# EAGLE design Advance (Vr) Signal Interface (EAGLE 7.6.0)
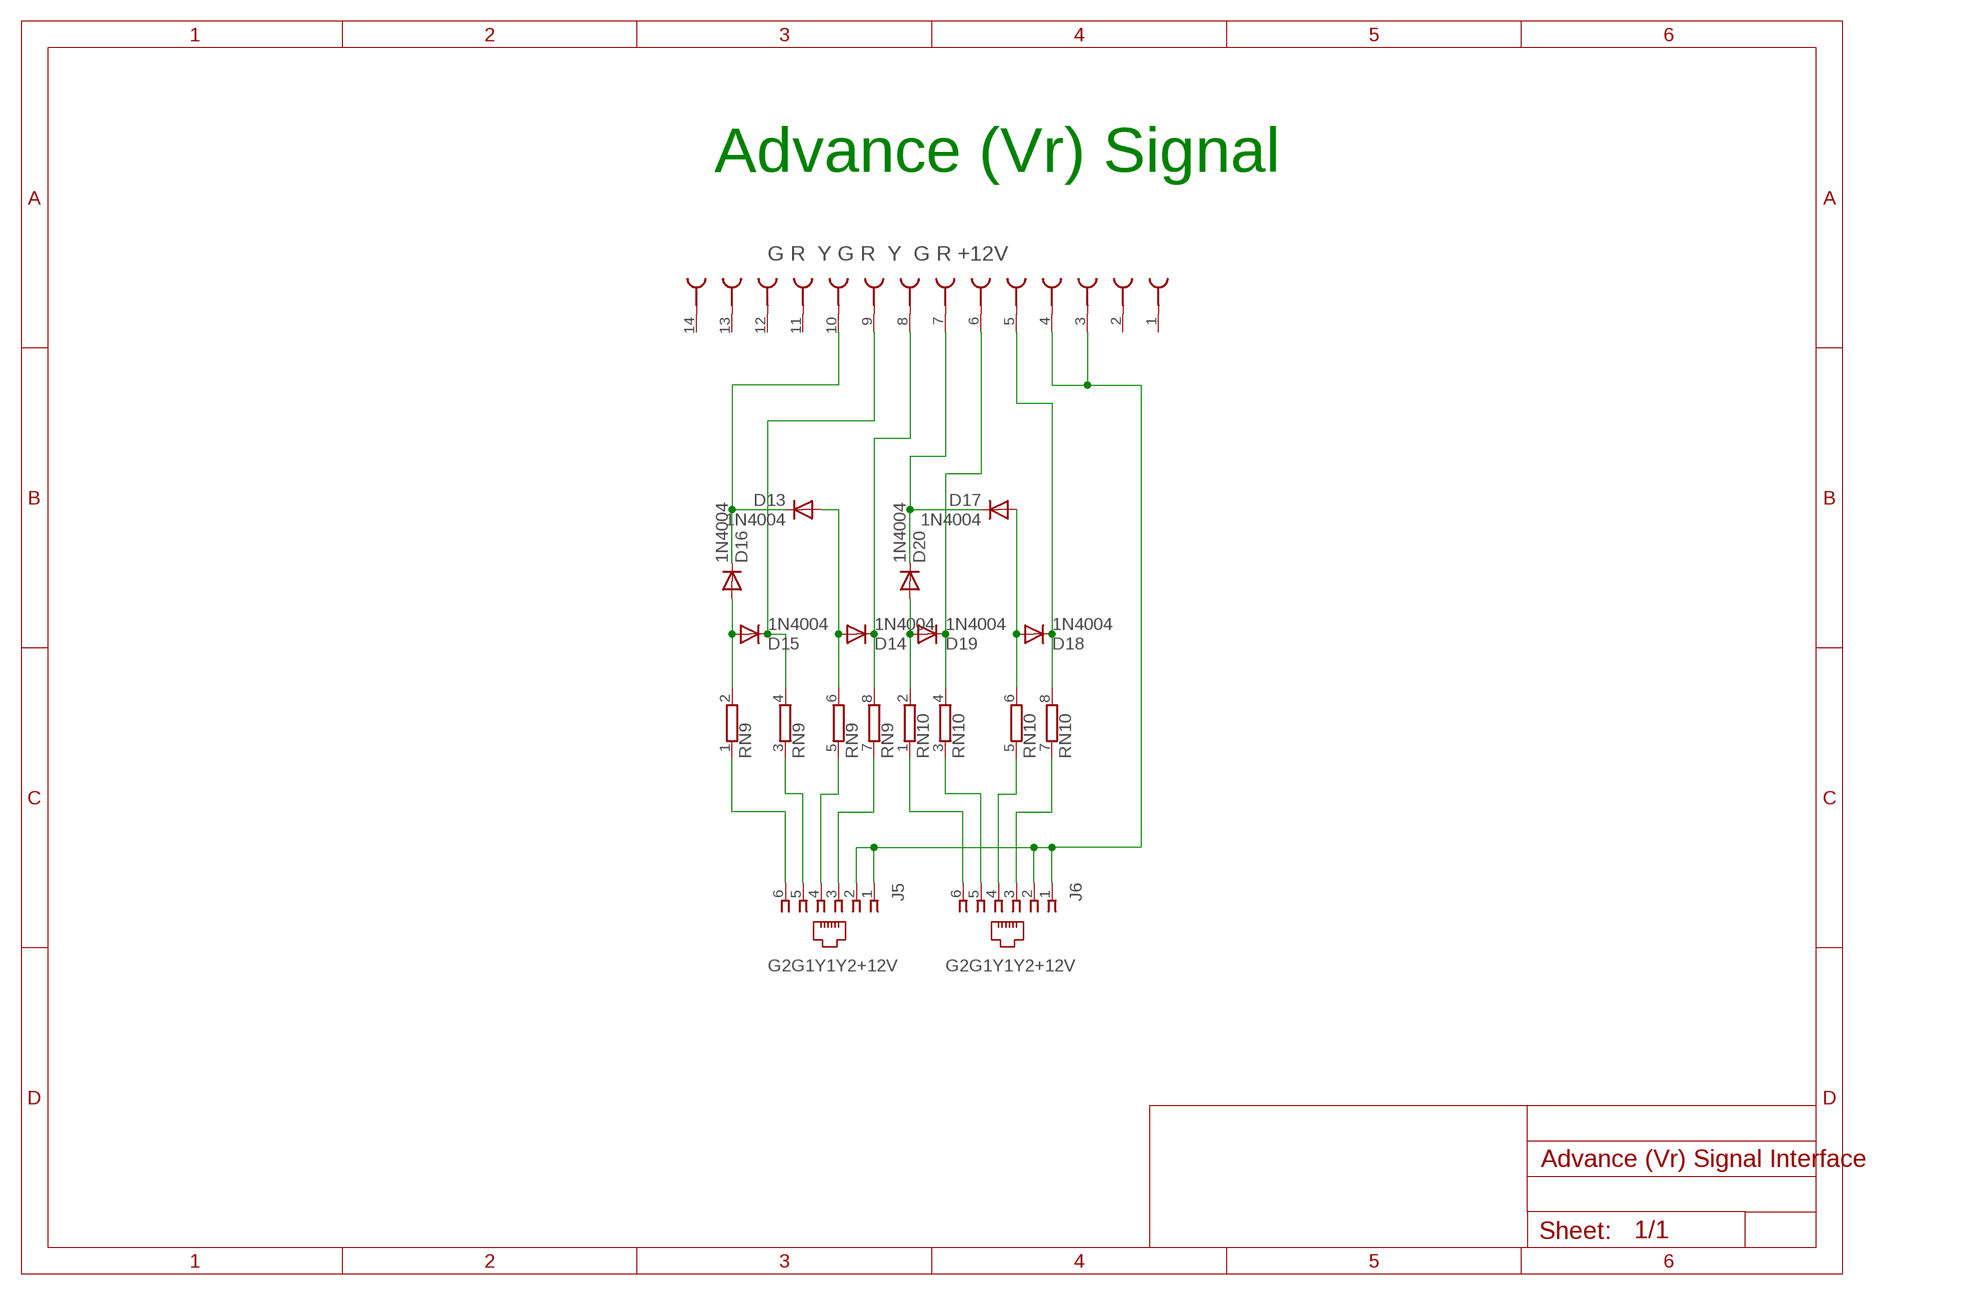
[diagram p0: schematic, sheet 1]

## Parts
D13  1N4004  [DO41-10]
D14  1N4004  [DO41-10]
D15  1N4004  [DO41-10]
D16  1N4004  [DO41-10]
D17  1N4004  [DO41-10]
D18  1N4004  [DO41-10]
D19  1N4004  [DO41-10]
D20  1N4004  [DO41-10]
J5  520250-3  [520250-3]
J6  520250-3  [520250-3]
RN9  E4RP  [SIL8]
RN10  E4RP  [SIL8]
U$11  AMP_FEMALE_PLUG  [AMP_FEMALE_PLUG]

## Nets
N$47: J5.3 RN9.7
N$48: D13.C D16.C U$11.10(SK9)
N$49: D13.A D14.A RN9.6
N$50: D15.A D16.A RN9.2
N$51: D14.C RN9.8 U$11.8(SK7)
N$52: D15.C RN9.4 U$11.9(SK8)
N$53: J5.4 RN9.5
N$54: J5.5 RN9.3
N$55: J5.6 RN9.1
N$56: J5.1 J5.2 J6.1 J6.2 U$11.3(SK2) U$11.4(SK3)
N$57: D18.C RN10.8 U$11.5(SK4)
N$58: J6.4 RN10.5
N$59: J6.5 RN10.3
N$60: J6.6 RN10.1
N$61: J6.3 RN10.7
N$62: D19.A D20.A RN10.2
N$63: D19.C RN10.4 U$11.6(SK5)
N$64: D17.C D20.C U$11.7(SK6)
N$84: D17.A D18.A RN10.6
Unconnected: U$11.1(SK) U$11.2(SK1) U$11.11(SK10) U$11.12(SK11) U$11.13(SK12) U$11.14(SK13)

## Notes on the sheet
- Advance (Vr) Signal
- G R  Y G R  Y  G R +12V
- G2G1Y1Y2+12V | G2G1Y1Y2+12V

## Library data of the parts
D13-D20 = diode:1N4004: DIODE
J5 J6 = con-amp:520250-3: AMP connector; MF: TYCO ELECTRONICS; MPN: 5520250-3; OC_FARNELL: unknown; OC_NEWARK: 42K8724
RN9 RN10 = resistor-sil:E4RP: SIL RESISTOR; OC_FARNELL: unknown; OC_NEWARK: unknown
U$11 = con-3m:AMP_FEMALE_PLUG

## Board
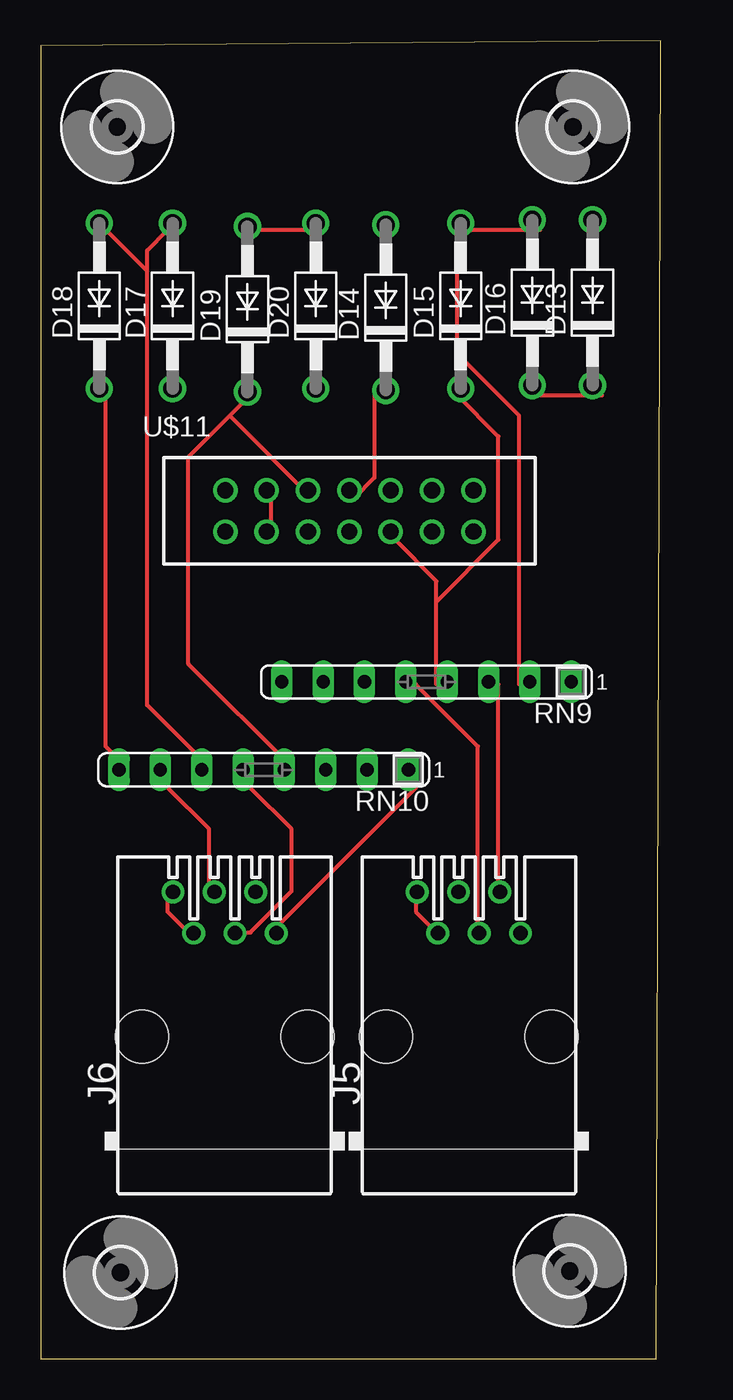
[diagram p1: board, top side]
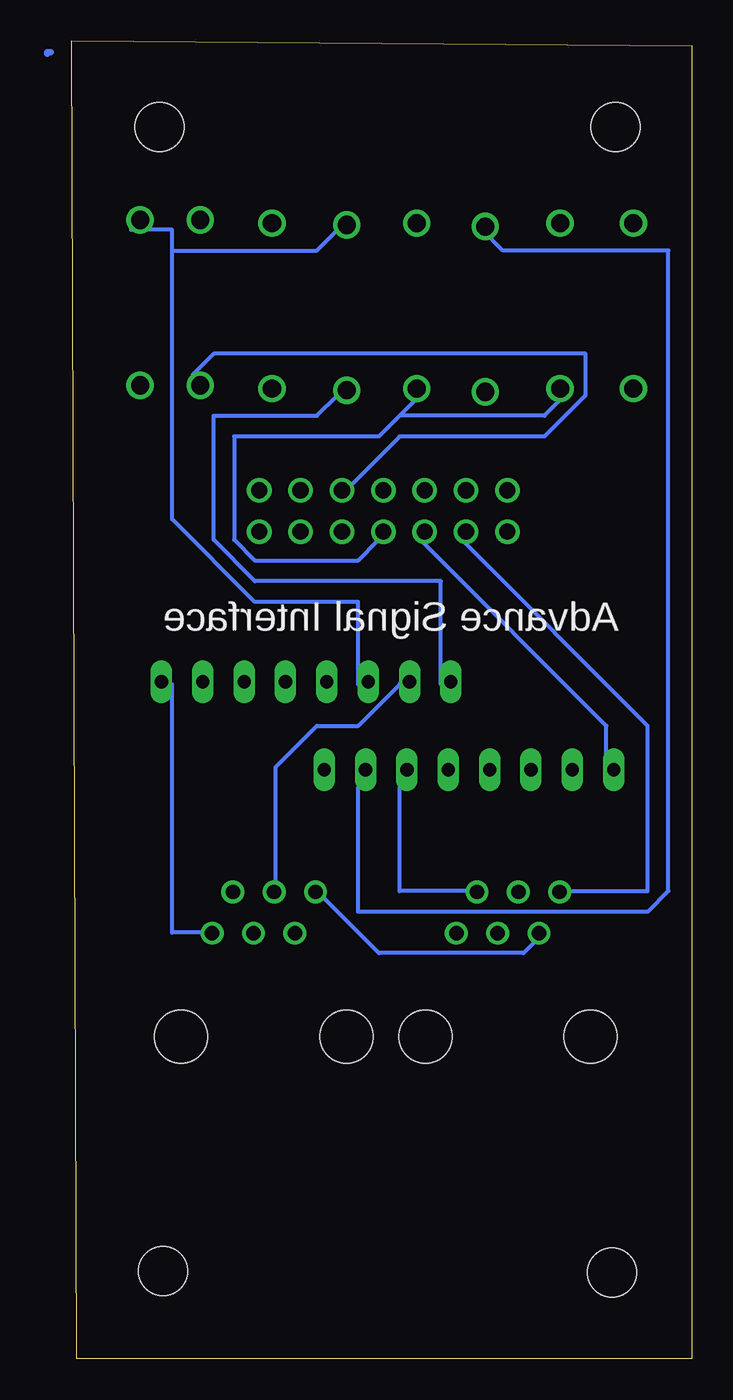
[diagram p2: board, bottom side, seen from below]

Size 38.1 x 81 mm. Coordinates in mm from the lower left corner, seen from the top.
Outline: 0,0 37.8,0 38.1,81 0,80.7 0,0
Copper layers (1*16): Top 0.035mm / dielectric 1.5mm / Bottom 0.035mm
Design rules "default": minimum track width 10mil, minimum drill 24mil, track to track 8mil, track to pad 8mil, pad to pad 8mil, via to via 8mil, smd to smd 8mil, copper to edge 40mil, drill to drill 8mil, minimum pad ring 10mil, minimum via ring 8mil, stop-mask expansion 4mil, vias tented up to drill 0mil, thermal gap 10mil

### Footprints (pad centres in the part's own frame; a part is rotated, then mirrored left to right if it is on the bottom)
DO41-10 = drill 1.118: A 5.08,0; C -5.08,0
520250-3 = drill 0.889: 1 -3.175,8.89; 2 -1.905,6.35; 3 -0.635,8.89; 4 0.635,6.35; 5 1.905,8.89; 6 3.175,6.35 | hole 3.251: -5.08,0; 5.08,0
SIL8 = drill 0.813 long: 1 -8.89,0; 2 -6.35,0; 3 -3.81,0; 4 -1.27,0; 5 1.27,0; 6 3.81,0; 7 6.35,0; 8 8.89,0
AMP_FEMALE_PLUG = drill 1 pad 1.422: 1 -10.16,-1.27; 2 -10.16,1.27; 3 -7.62,-1.27; 4 -7.62,1.27; 5 -5.08,-1.27; 6 -5.08,1.27; 7 -2.54,-1.27; 8 -2.54,1.27; 9 0,-1.27; 10 0,1.27; 11 2.54,-1.27; 12 2.54,1.27; 13 5.08,-1.27; 14 5.08,1.27
3,0 = hole 3: 0,0

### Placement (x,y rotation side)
D13  33.9,64.9 90 top
D14  21.2,64.6 90 top
D15  25.8,64.7 90 top
D16  30.2,64.9 90 top
D17  8.1,64.7 90 top
D18  3.6,64.7 90 top
D19  12.7,64.5 90 top
D20  16.9,64.7 90 top
J5  26.3,19.8 0 top
J6  11.3,19.8 0 top
RN9  23.7,41.6 180 top
RN10  13.7,36.2 180 top
U$11  21.5,52.1 0 top
U$12  [3,0]  4.7,75.7 0 top
U$13  [3,0]  32.7,75.7 0 top
U$14  [3,0]  4.9,5.3 0 top
U$15  [3,0]  32.5,5.4 0 top

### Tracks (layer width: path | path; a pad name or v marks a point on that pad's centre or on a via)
N$47
  Bottom 0.254: RN9.7 17.96,41.44 20.5,38.9 23.04,38.9 25.58,36.36 25.58,28.74 J5.3
N$48
  Top 0.254: D13.C 34.47,59.22 30.66,59.22 D16.C
  Bottom 0.254: U$11.10 21.77,52.87 17.96,56.68 9.07,56.68 6.53,59.22 6.53,61.76 29.39,61.76 30.66,60.49 D16.C
N$49
  Bottom 0.254: 31.93,68.11 31.93,69.38 34.47,69.38 D13.A | 31.93,68.11 31.93,51.6 26.85,46.52 20.5,46.52 20.5,41.44 RN9.6 | 31.93,68.11 23.04,68.11 21.77,69.38 D14.A
N$50
  Top 0.254: 25.58,69.38 25.58,61.76 29.39,57.95 29.39,41.44 RN9.2 | 25.58,69.38 30.66,69.38 D16.A | 25.58,69.38 D15.A
N$51
  Top 0.254: U$11.8 19.23,52.87 20.5,54.14 20.5,59.22 D14.C
  Bottom 0.254: RN9.8 15.42,41.44 15.42,47.79 26.85,47.79 29.39,50.33 29.39,57.95 23.04,57.95 21.77,59.22 D14.C
N$52
  Top 0.254: 24.31,46.52 24.31,47.79 21.77,50.33 U$11.9 | 24.31,46.52 24.31,41.44 RN9.4 | 24.31,46.52 28.12,50.33 28.12,56.68 25.58,59.22 D15.C
N$53
  Top 0.254: RN9.5 23.04,41.44 26.85,37.63 26.85,26.2 J5.4
N$54
  Top 0.254: RN9.3 28.12,41.44 28.12,28.74 J5.5
N$55
  Bottom 0.254: RN9.1 31.93,41.44 31.93,26.2 29.39,26.2 J5.6
N$56
  Top 0.254: J5.2 24.31,26.2 23.04,27.47 23.04,28.74 J5.1 | U$11.3 14.15,50.33 14.15,52.87 U$11.4 | J6.2 9.07,26.2 7.8,27.47 7.8,28.74 J6.1
  Bottom 0.254: U$11.3 14.15,50.33 2.72,38.9 2.72,28.74 7.8,28.74 J6.1 | J5.1 23.04,28.74 19.23,24.93 10.34,24.93 9.07,26.2 J6.2
N$57
  Top 0.254: RN10.8 5.26,36.36 3.99,37.63 3.99,59.22 D18.C
  Bottom 0.254: U$11.5 16.69,50.33 5.26,38.9 5.26,36.36 RN10.8
N$58
  Top 0.254: RN10.5 12.88,35.09 15.42,32.55 15.42,28.74 12.88,26.2 11.61,26.2 J6.4
N$59
  Bottom 0.254: RN10.3 17.96,35.09 17.96,28.74 12.88,28.74 J6.5
N$60
  Top 0.254: RN10.1 23.04,35.09 14.15,26.2 J6.6
N$61
  Top 0.254: RN10.7 7.8,35.09 10.34,32.55 10.34,28.74 J6.3
N$62
  Top 0.254: D20.A 16.69,69.38 12.88,69.38 D19.A
  Bottom 0.254: RN10.2 20.5,35.09 20.5,27.47 2.72,27.47 1.45,28.74 1.45,68.11 11.61,68.11 12.88,69.38 D19.A
N$63
  Top 0.254: 11.61,57.95 12.88,59.22 D19.C | 11.61,57.95 9.07,55.41 9.07,42.71 15.42,36.36 RN10.4 | 11.61,57.95 16.69,52.87 U$11.6
N$64
  Bottom 0.254: 17.96,57.95 16.69,59.22 D20.C | 17.96,57.95 19.23,56.68 28.12,56.68 28.12,50.33 26.85,49.06 20.5,49.06 19.23,50.33 U$11.7 | 17.96,57.95 9.07,57.95 7.8,59.22 D17.C
N$83
  Bottom 0.406: 39.4,80.3 39.6,80.3 39.6,80.2
N$84
  Top 0.254: 6.53,66.84 6.53,68.11 7.8,69.38 D17.A | 6.53,66.84 6.53,40.17 10.34,36.36 RN10.6 | 6.53,66.84 3.99,69.38 D18.A

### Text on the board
bPlace: Advance Signal Interface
